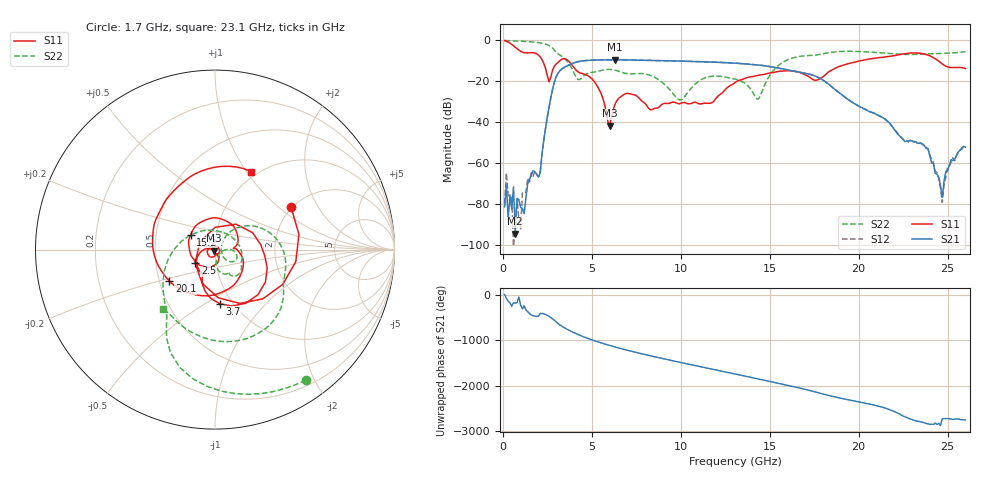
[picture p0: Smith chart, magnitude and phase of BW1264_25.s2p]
!Keysight Technologies,N5245B,MY57181159,A.13.60.06
!Date: Friday, December 18, 2020 23:53:15
!Correction: S11(Full 2 Port(1,2))
!S21(Full 2 Port(1,2))
!S12(Full 2 Port(1,2))
!S22(Full 2 Port(1,2))
!S2P File: Measurements: S11, S21, S12, S22:
# Hz S  dB  R 50
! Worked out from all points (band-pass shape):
!   260 points, 100 MHz to 26 GHz, reference 50 ohm
!   highest |S21| = -9.73 dB at 6.3 GHz (marker M1); lowest = -94.6 dB at 700 MHz (marker M2)
!   |S21| within 3 dB of the highest: 3.599 GHz to 14.77 GHz (11.17 GHz wide, 122 % of centre)
!   lowest |S11| = -41.9 dB at 6 GHz (marker M3), VSWR 1.02, Z = 49.6 - j0.664 ohm
!   |S11| at or under -10 dB: 2.221 GHz to 3.231 GHz (1.01 GHz wide, 37 % of centre); 3.647 GHz to 20.23 GHz (16.59 GHz wide, 139 % of centre); 24.44 GHz to end of sweep
!   |S22| runs from -29.3 to -0.3 dB; largest |S21 - S12| = 0.00059
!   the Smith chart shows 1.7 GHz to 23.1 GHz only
!   S11 on the Smith chart (normalised r, x): 1.7 GHz: 1.96, +1.22; 2.5 GHz: 0.79, -0.12; 3.7 GHz: 0.87, -0.58; 15.2 GHz: 0.75, +0.13; 20.1 GHz: 0.56, -0.22; 23.1 GHz: 0.93, +1.05
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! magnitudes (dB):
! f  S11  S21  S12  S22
! 100 MHz  -0.4  -81.4  -79.9  -0.3
! 200 MHz  -0.7  -70.7  -65.0  -0.4
! 700 MHz  -3.6  -94.6  -88.2  -0.5
! 1.7 GHz  -6.3  -63.9  -66.6  -1.1
! 2.1 GHz  -8.3  -64.9  -64.3  -1.5
! 2.5 GHz  -17.5  -37.7  -37.8  -2.4
! 3.7 GHz  -10.4  -12.3  -12.3  -11.4
! 4.5 GHz  -16.5  -10.2  -10.2  -17.9
! 6 GHz  -41.9  -9.7  -9.7  -14.4
! 6.3 GHz  -31.6  -9.7  -9.7  -14.8
! 8.8 GHz  -32.7  -10.1  -10.1  -19.7
! 13.1 GHz  -20.6  -11.4  -11.4  -19.2
! 14.3 GHz  -17.4  -12.2  -12.2  -29.0
! 15.2 GHz  -16.0  -13.3  -13.3  -15.1
! 17.4 GHz  -19.2  -17.2  -17.2  -7.6
! 20.1 GHz  -10.2  -32.8  -32.9  -5.7
! 21.7 GHz  -8.1  -40.3  -40.3  -6.6
! 23.1 GHz  -6.4  -49.9  -49.6  -7.1
! 23.9 GHz  -7.5  -53.2  -53.3  -6.8
! 24.7 GHz  -11.7  -77.0  -79.3  -6.6
! 25 GHz  -13.2  -64.0  -62.0  -6.5
! 26 GHz  -14.0  -52.3  -51.7  -5.7
